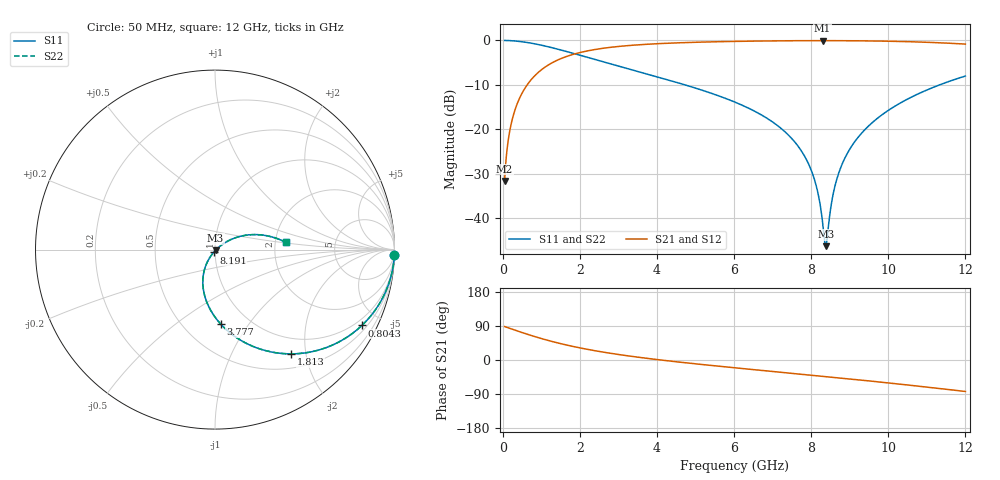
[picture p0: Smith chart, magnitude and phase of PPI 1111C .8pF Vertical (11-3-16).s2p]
# GHz S MA R 50
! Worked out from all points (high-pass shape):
!   1601 points, 50 MHz to 12 GHz, reference 50 ohm
!   highest |S21| = -0.05 dB at 8.296 GHz (marker M1); lowest = -31.7 dB at 50 MHz (marker M2)
!   |S21| within 3 dB of the highest: 1.865 GHz to end of sweep
!   lowest |S11| = -46.4 dB at 8.378 GHz (marker M3), VSWR 1.01, Z = 50.3 - j0.338 ohm
!   |S11| at or under -10 dB: 4.723 GHz to 11.34 GHz (6.613 GHz wide, 82.4 % of centre)
!   |S22| runs from -46.4 to 0.0 dB; largest |S21 - S12| = 0
!   S11 on the Smith chart (normalised r, x): 50 MHz: 1, -65; 804.3 MHz: 0.72, -3.99; 1.813 GHz: 0.72, -1.73; 3.777 GHz: 0.75, -0.75; 8.191 GHz: 0.98, -0.03; 12 GHz: 2.29, +0.22
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0.05  0.9997 -1.8  0.02614 88.2  0.02614 88.2  0.9997 -1.8
0.1695  0.9961 -6.0  0.08831 84.0  0.08831 84.0  0.9961 -6.0
0.3039375  0.9876 -10.7  0.157 79.3  0.157 79.3  0.9876 -10.7
0.5130625  0.9657 -17.9  0.2594 72.1  0.2594 72.1  0.9657 -17.9
0.8043438  0.9211 -27.3  0.3887 62.7  0.3887 62.7  0.9211 -27.3
1.812625  0.7189 -53.9  0.6938 36.0  0.6938 36.0  0.7189 -53.9
2.044156  0.6738 -58.8  0.7374 31.1  0.7374 31.1  0.6738 -58.8
3.776906  0.4149 -85.7  0.9073 3.9  0.9073 3.9  0.4149 -85.7
4.038312  0.3856 -88.9  0.92 0.7  0.92 0.7  0.3856 -88.9
6.025  0.2016 -109.6  0.9757 -20.6  0.9757 -20.6  0.2016 -109.6
7.324562  0.09313 -120.8  0.9911 -33.3  0.9911 -33.3  0.09313 -120.8
7.735344  0.05782 -123.0  0.9935 -37.3  0.9935 -37.3  0.05782 -123.0
8.019156  0.03291 -122.2  0.9945 -40.1  0.9945 -40.1  0.03291 -122.2
8.190938  0.01776 -116.6  0.9947 -41.8  0.9947 -41.8  0.01776 -116.6
8.2955  0.008965 -101.0  0.9948 -42.9  0.9948 -42.9  0.008965 -101.0
8.377656  0.004796 -44.4  0.9948 -43.7  0.9948 -43.7  0.004796 -44.4
8.422469  0.006321 -3.9  0.9947 -44.1  0.9947 -44.1  0.006321 -3.9
8.609188  0.0221 31.0  0.9943 -46.0  0.9943 -46.0  0.0221 31.0
8.878063  0.04753 35.0  0.9933 -48.7  0.9933 -48.7  0.04753 35.0
9.333656  0.09264 33.2  0.9897 -53.4  0.9897 -53.4  0.09264 33.2
10.01331  0.1641 27.3  0.9799 -60.6  0.9799 -60.6  0.1641 27.3
12  0.397 5.8  0.9095 -83.1  0.9095 -83.1  0.397 5.8
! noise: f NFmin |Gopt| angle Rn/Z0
0.05  0.001128  0.9743  1.627  0.00998
1.372  0.0046  0.7372  11.45  0.003467
2.701  0.007416  0.6828  17.72  0.004426
4.031  0.01  0.657  24.1  0.00533
5.36  0.01253  0.6452  30.36  0.006251
6.682  0.01509  0.6428  36.37  0.00725
8.012  0.01781  0.6476  42.16  0.008405
9.341  0.02077  0.6583  47.68  0.00979
10.67  0.02406  0.674  52.94  0.01151
12  0.02782  0.6938  57.97  0.01369
